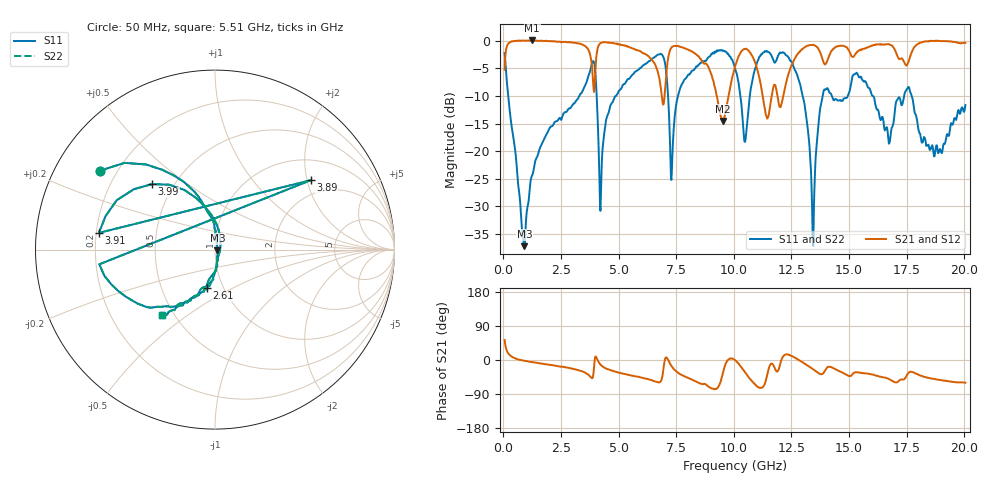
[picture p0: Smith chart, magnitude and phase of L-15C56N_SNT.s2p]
#	mhz	s	ma	r	50
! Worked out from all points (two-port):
!   1001 points, 50 MHz to 20.05 GHz, reference 50 ohm
!   highest |S21| = 0.08 dB at 1.25 GHz (marker M1); lowest = -14.5 dB at 9.53 GHz (marker M2)
!   |S21| within 3 dB of the highest: 78.06 MHz to 3.783 GHz (3.705 GHz wide, 192 % of centre); 17.64 GHz to end of sweep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
!   lowest |S11| = -37.2 dB at 910 MHz (marker M3), VSWR 1.03, Z = 51.3 - j0.373 ohm
!   |S11| at or under -10 dB: 206.8 MHz to 3.288 GHz (3.081 GHz wide, 176 % of centre); 16.03 GHz to 17.39 GHz (1.362 GHz wide, 8.15 % of centre); 17.72 GHz to end of sweep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
!   |S22| runs from -37.2 to -1.7 dB; largest |S21 - S12| = 0
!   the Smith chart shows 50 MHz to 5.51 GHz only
!   S11 on the Smith chart (normalised r, x): 50 MHz: 0.14, +0.31; 2.61 GHz: 0.84, -0.38; 3.89 GHz: 1.54, +2.10; 3.91 GHz: 0.21, +0.07; 3.99 GHz: 0.38, +0.37; 5.51 GHz: 0.43, -0.40
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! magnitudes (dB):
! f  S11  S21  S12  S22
! 50 MHz  -2.2  -5.2  -5.2  -2.2
! 910 MHz  -37.2  0.1  0.1  -37.2
! 1.25 GHz  -24.4  0.1  0.1  -24.4
! 2.61 GHz  -13.2  -0.2  -0.2  -13.2
! 3.39 GHz  -9.4  -0.6  -0.6  -9.4
! 3.89 GHz  -3.6  -7.4  -7.4  -3.6
! 3.91 GHz  -3.7  -8.6  -8.6  -3.7
! 3.99 GHz  -5.9  -5.4  -5.4  -5.9
! 4.23 GHz  -27.8  -0.4  -0.4  -27.8
! 5.51 GHz  -6.6  -1.2  -1.2  -6.6
! 6.73 GHz  -2.5  -6.1  -6.1  -2.5
! 7.31 GHz  -23.5  -1.1  -1.1  -23.5
! 7.77 GHz  -7.7  -1.2  -1.2  -7.7
! 9.53 GHz  -1.8  -14.5  -14.5  -1.8
! 10.05 GHz  -4.9  -4.6  -4.6  -4.9
! 10.49 GHz  -18.3  -1.5  -1.5  -18.3
! 11.45 GHz  -2.0  -14.1  -14.1  -2.0
! 12.45 GHz  -3.6  -5.0  -5.0  -3.6
! 13.39 GHz  -29.2  -0.7  -0.7  -29.2
! 13.99 GHz  -8.8  -4.2  -4.2  -8.8
! 16.73 GHz  -18.7  -0.6  -0.6  -18.7
! 20.05 GHz  -11.6  -0.3  -0.3  -11.6
